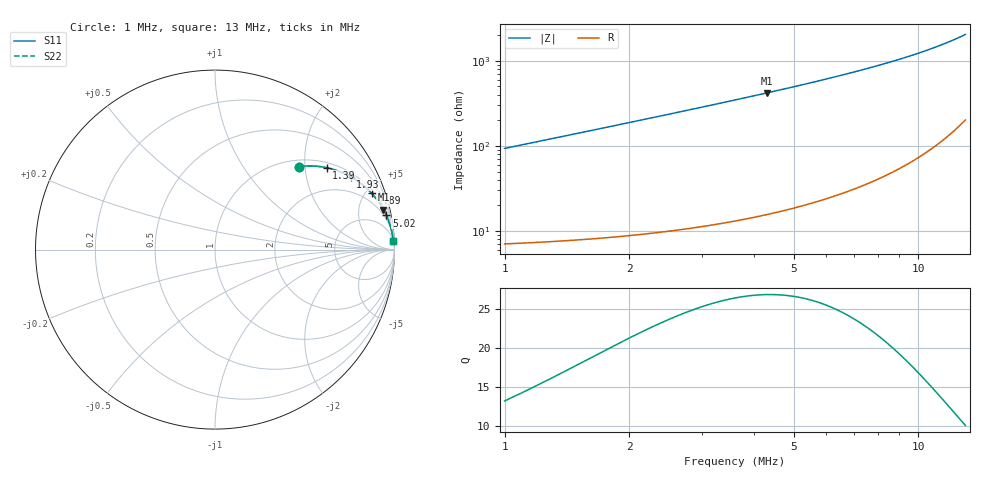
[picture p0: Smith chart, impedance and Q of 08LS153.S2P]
! Coilcraft 0805LS-153 Chip Inductor
! 18 September 2002
# MHZ S MA R 50
!Freq  MagS11  AngS11  MagS21  AngS21  MagS12  AngS12  MagS22  AngS22
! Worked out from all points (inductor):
!   401 points, 1 MHz to 13 MHz, reference 50 ohm
!   read as one part in series: L = 14.9 uH near 1.06 MHz
!   highest Q = 26.8 at 4.3 MHz (marker M1), where L = 15.5 uH
!   S11 on the Smith chart (normalised r, x): 1 MHz: 1.14, +1.86; 1.39 MHz: 1.15, +2.60; 1.93 MHz: 1.17, +3.62; 2.89 MHz: 1.22, +5.48; 5.02 MHz: 1, +10; 13 MHz: 5, +41
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1  0.6585 44.6  0.7044 -41.0  0.7044 -41.0  0.6585 44.6
1.06  0.6797 43.2  0.686 -42.7  0.686 -42.7  0.6797 43.2
1.18  0.7176 40.5  0.6504 -45.7  0.6504 -45.7  0.7176 40.5
1.39  0.7711 36.3  0.5928 -50.3  0.5928 -50.3  0.7711 36.3
1.51  0.7958 34.2  0.5628 -52.6  0.5628 -52.6  0.7958 34.2
1.66  0.8218 31.8  0.5282 -55.2  0.5282 -55.2  0.8218 31.8
1.78  0.8395 30.1  0.5027 -57.0  0.5027 -57.0  0.8395 30.1
1.93  0.8584 28.2  0.4735 -59.0  0.4735 -59.0  0.8584 28.2
2.14  0.8799 25.9  0.4369 -61.5  0.4369 -61.5  0.8799 25.9
2.38  0.8992 23.6  0.4004 -63.9  0.4004 -63.9  0.8992 23.6
2.62  0.9143 21.6  0.3688 -66.0  0.3688 -66.0  0.9143 21.6
2.89  0.9277 19.7  0.338 -68.0  0.338 -68.0  0.9277 19.7
3.01  0.9327 19.0  0.3257 -68.7  0.3257 -68.7  0.9327 19.0
3.58  0.9506 16.0  0.2766 -71.8  0.2766 -71.8  0.9506 16.0
4.3  0.9646 13.3  0.2304 -74.6  0.2304 -74.6  0.9646 13.3
5.02  0.9733 11.3  0.1958 -76.6  0.1958 -76.6  0.9733 11.3
5.95  0.9805 9.3  0.162 -78.4  0.162 -78.4  0.9805 9.3
7  0.9854 7.7  0.1334 -79.9  0.1334 -79.9  0.9854 7.7
7.96  0.9884 6.5  0.1131 -80.9  0.1131 -80.9  0.9884 6.5
9.01  0.9905 5.4  0.09505 -81.6  0.09505 -81.6  0.9905 5.4
11.02  0.9929 3.9  0.06854 -82.1  0.06854 -82.1  0.9929 3.9
13  0.994 2.8  0.04883 -81.5  0.04883 -81.5  0.994 2.8
